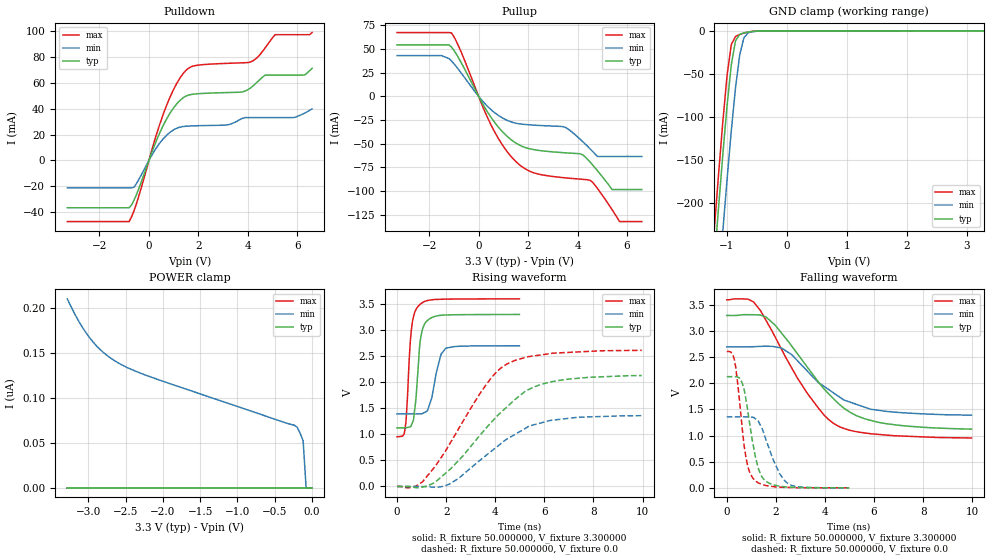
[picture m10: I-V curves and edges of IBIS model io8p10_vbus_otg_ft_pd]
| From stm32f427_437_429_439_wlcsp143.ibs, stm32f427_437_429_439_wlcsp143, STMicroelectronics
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|   Model io8p10_vbus_otg_ft_pd
[Model]  io8p10_vbus_otg_ft_pd
Model_type I/O
Polarity   Non-Inverting
Enable   Active-Low
Vinl =   0.990000V
Vinh =   2.310000V
Vmeas =  1.650000V
Cref =   40.000000pF
Rref =   100.000000M
Vref =   0.0V
C_comp   3.304800pF   3.199300pF   3.429300pF
[Temperature Range]   25.000000   0.125000k   -40.000000
[Pullup Reference]   3.300000V   2.700000V   3.600000V
[Pulldown Reference]   0.0V   0.0V   0.0V
[POWER Clamp Reference]   3.300000V   2.700000V   3.600000V
[GND Clamp Reference]   0.0V   0.0V   0.0V
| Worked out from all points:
|   slope of the pulldown table from 0 to 0.495 V, typ, clamps not added: 20.9 ohm
|   slope of the pullup table from 0 to 0.495 V, typ, clamps not added: 22.6 ohm
|   GND clamp passes 1 mA (typ) near -0.61 V on its own axis
|   rising waveform, R_fixture 50.000000, V_fixture 3.300000: 20-80 % time 228ps typ, 355ps min, 207ps max; typ from 1.12 V to 3.3 V
|   rising waveform, R_fixture 50.000000, V_fixture 0.0: 20-80 % time 2.54ns typ, 2.33ns min, 2.1ns max; typ from 0 V to 2.13 V
|   falling waveform, R_fixture 50.000000, V_fixture 3.300000: 20-80 % time 2.29ns typ, 2.07ns min, 2.05ns max; typ from 3.3 V to 1.12 V
|   falling waveform, R_fixture 50.000000, V_fixture 0.0: 20-80 % time 480ps typ, 676ps min, 387ps max; typ from 2.13 V to 0 V
[Pulldown]
|Voltage   I(typ)   I(min)   I(max)
-3.3V     -36.41mA   -21.08mA   -47.03mA
-800mV    -36.41mA   -21.08mA   -47.03mA
-600mV    -30.48mA   -20.53mA   -38.65mA
700mV     31.4mA     19.11mA    41.71mA
1.2V      45.15mA    25.37mA    61.75mA
1.6V      50.35mA    26.5mA     71.06mA
3.1V      52.27mA    27.26mA    74.75mA
4.1V      55.7mA     32.99mA    75.8mA
4.7V      65.72mA    32.99mA    86.69mA
5.1V      65.72mA    32.99mA    96.9mA
6.3V      65.87mA    36.5mA     96.9mA
6.6V      70.93mA    39.71mA    98.5mA
[Pullup]
|Voltage   I(typ)   I(min)   I(max)
-3.3V     54.22mA    42.91mA    67.18mA
-1.1V     51.99mA    37.29mA    66.9mA
500mV     -22.07mA   -14mA      -30.03mA
1.5V      -49.1mA    -28.3mA    -68.56mA
2.2V      -56.04mA   -30.32mA   -80.35mA
3.5V      -59.53mA   -32.66mA   -85.92mA
4.2V      -61.44mA   -47.49mA   -87.46mA
4.5V      -69.06mA   -55.13mA   -88.4mA
4.8V      -78.22mA   -63.4mA    -96.84mA
5.4V      -98.3mA    -63.4mA    -119.6mA
5.7V      -98.3mA    -63.4mA    -132mA
6.6V      -98.3mA    -63.4mA    -132mA
[GND_clamp]
|Voltage   I(typ)   I(min)   I(max)
-3.3V     -2.319A    -2.398A    -2.292A
-1.2V     -265.6mA   -356.2mA   -227.3mA
-1.13V    -202.8mA   -293mA     -164.3mA
-1.06V    -142.3mA   -231.2mA   -104.3mA
-990mV    -86.15mA   -171.7mA   -51.01mA
-920mV    -39.05mA   -115.6mA   -15.73mA
-850mV    -11.41mA   -65.74mA   -6.38mA
-780mV    -4.058mA   -27.6mA    -4.167mA
-710mV    -2.296mA   -7.89mA    -2.605mA
-640mV    -1.302mA   -2.283mA   -1.381mA
-570mV    -629.1uA   -918.9uA   -580.8uA
3.28V     81.28uA    57.87uA    93.98uA
[POWER_clamp]
|Voltage   I(typ)   I(min)   I(max)
-3.28V    0A         210.1nA    0A
-3.12V    0A         184.2nA    0A
-2.96V    0A         164.6nA    0A
-2.8V     0A         150.7nA    0A
-2.6V     0A         139nA      0A
-2.16V    0A         123.2nA    0A
-240mV    0A         69.7nA     0A
-200mV    0A         67.32nA    0A
-160mV    0A         60.72nA    0A
-120mV    0A         52.23nA    0A
-80mV     0A         0A         0A
0V        0A         0A         0A
[Ramp]
| variable   typ   min   max
dV/dt_r  1.26648/2.53268n   0.81072/2.32748n   1.56420/2.10306n
dV/dt_f  1.28250/2.27218n   0.77550/2.05246n   1.57454/2.04776n
R_load = 50.000000
[Rising Waveform]
R_fixture= 50.000000
V_fixture= 3.300000
V_fixture_min= 2.700000
V_fixture_max= 3.600000
|time   V(typ)   V(min)   V(max)
0s        1.123V     1.391V     954mV
300.3ps   1.125V     1.391V     1.025V
370.4ps   1.127V     1.391V     1.281V
580.6ps   1.172V     1.391V     2.989V
670.7ps   1.281V     1.39V      3.258V
850.9ps   2.209V     1.391V     3.45V
940.9ps   2.771V     1.393V     3.492V
1.111ns   3.107V     1.417V     3.545V
1.992ns   3.288V     2.653V     3.593V
4.985ns   3.299V     2.699V     3.598V
[Rising Waveform]
R_fixture= 50.000000
V_fixture= 0.0
V_fixture_min= 0.0
V_fixture_max= 0.0
|time   V(typ)   V(min)   V(max)
0s        344.2uV    194.9uV    668.6uV
460.5ps   -2.446mV   135.8uV    -26.63mV
1.041ns   -9.915mV   -1.885mV   90.36mV
1.522ns   70.99mV    -16.19mV   367.3mV
2.142ns   321.3mV    47.41mV    812.9mV
3.604ns   1.107V     586.4mV    1.936V
4.444ns   1.512V     898.8mV    2.338V
5.205ns   1.819V     1.108V     2.471V
6.166ns   1.994V     1.256V     2.544V
9.97ns    2.127V     1.357V     2.611V
[Falling Waveform]
R_fixture= 50.000000
V_fixture= 3.300000
V_fixture_min= 2.700000
V_fixture_max= 3.600000
|time   V(typ)   V(min)   V(max)
0s        3.299V     2.699V     3.598V
1.081ns   3.313V     2.7V       3.561V
1.602ns   3.269V     2.709V     3.204V
2.242ns   2.956V     2.673V     2.642V
3.303ns   2.297V     2.225V     1.795V
3.984ns   1.883V     1.936V     1.383V
4.484ns   1.643V     1.773V     1.196V
5.265ns   1.385V     1.601V     1.077V
6.246ns   1.248V     1.481V     1.02V
9.97ns    1.123V     1.391V     954mV
[Falling Waveform]
R_fixture= 50.000000
V_fixture= 0.0
V_fixture_min= 0.0
V_fixture_max= 0.0
|time   V(typ)   V(min)   V(max)
0s        2.127V     1.357V     2.611V
300.3ps   2.128V     1.357V     2.477V
460.5ps   2.116V     1.357V     1.942V
620.6ps   2.018V     1.357V     1.189V
850.9ps   1.49V      1.359V     428.3mV
1.111ns   734.6mV    1.342V     160mV
1.491ns   174.7mV    1.069V     58.89mV
2.142ns   34.07mV    282.7mV    13.05mV
2.452ns   16.65mV    96.87mV    8.588mV
4.985ns   344.2uV    194.9uV    668.6uV
